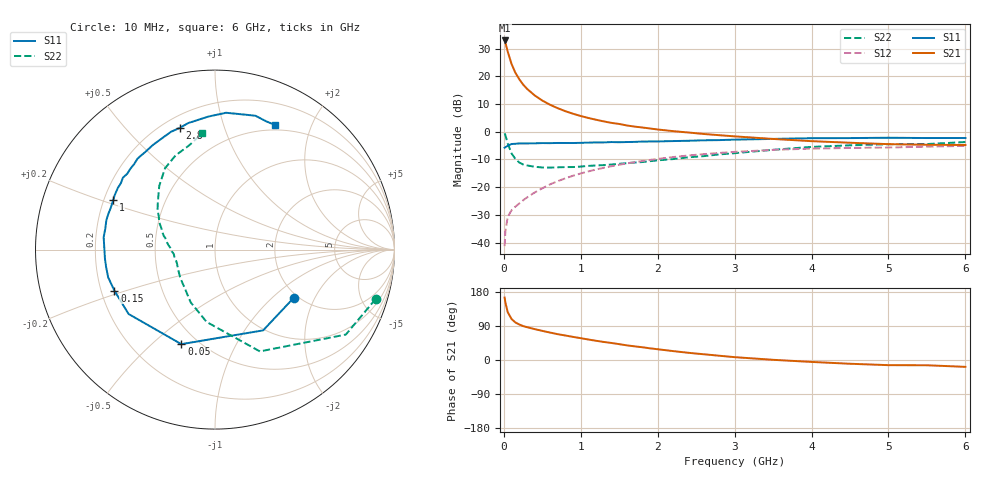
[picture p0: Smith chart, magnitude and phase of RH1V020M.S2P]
! SIEMENS Small Signal Semiconductors
! BFR106
! Si NPN RF Bipolar Junction Transistor in SOT23
! VCE = 1 V  IC = 20 mA
! Common Emitter S-Parameters:  August  1996
# GHz  S  MA  R  50
!  f  S11  S21  S12  S22
! GHz  MAG  ANG  MAG  ANG  MAG  ANG  MAG  ANG
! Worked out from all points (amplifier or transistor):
!   36 points, 10 MHz to 6 GHz, reference 50 ohm
!   highest |S21| = 33.0 dB at 10 MHz (marker M1)
!   |S21| within 3 dB of that: start of sweep to 40.81 MHz
!   unconditionally stable (mu >= 1): 332.5 MHz to 3.215 GHz; 4.097 GHz to end of sweep
!   at 250 MHz: K = 0.92, MSG = 20.9 dB, |S12| = -24.8 dB
!   at 1.4 GHz: K = 1.08, MAG = 6.0 dB, |S12| = -12.4 dB
!   at 6 GHz: K = 1.02, MAG = -0.8 dB, |S12| = -5.1 dB
!   S11 on the Smith chart (normalised r, x): 10 MHz: 1.89, -1.39; 50 MHz: 0.41, -0.62; 150 MHz: 0.25, -0.18; 1 GHz: 0.24, +0.22; 2.8 GHz: 0.27, +0.72; 6 GHz: 0.44, +1.50
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0.01  0.5142 -31.6  44.42 164.7  0.0086 79.8  0.9365 -17.1
0.02  0.5239 -59.2  40.78 152.0  0.0159 70.4  0.8692 -33.0
0.05  0.5592 -109.6  28.04 126.4  0.0291 51.9  0.6199 -66.2
0.1  0.6004 -143.3  16.75 108.1  0.0381 46.6  0.4059 -96.6
0.15  0.6053 -157.8  11.6 99.1  0.0445 49.0  0.3235 -114.8
0.2  0.6151 -165.5  8.879 93.8  0.0506 51.8  0.2787 -126.1
0.25  0.6143 -171.2  7.12 89.6  0.0578 54.4  0.2567 -136.0
0.3  0.6152 -175.3  5.975 86.7  0.0651 56.8  0.2469 -142.1
0.4  0.6177 178.2  4.535 81.5  0.0799 59.8  0.2331 -152.1
0.5  0.6242 173.6  3.652 76.9  0.0954 61.5  0.2263 -158.8
0.6  0.6223 169.2  3.071 72.4  0.1121 62.1  0.225 -163.0
0.7  0.6271 164.9  2.663 68.2  0.1281 62.0  0.228 -166.8
0.8  0.6267 161.6  2.347 64.6  0.1441 61.4  0.2301 -170.5
1  0.6305 154.2  1.922 57.6  0.1765 59.9  0.2349 -175.6
1.1  0.6362 151.2  1.77 54.0  0.1923 58.6  0.2418 -177.8
1.6  0.6519 136.3  1.297 38.6  0.2684 51.6  0.2708 171.3
2.2  0.6782 120.5  1.025 23.5  0.3491 41.9  0.3211 158.4
2.8  0.7061 106.1  0.866 11.3  0.4139 31.9  0.3896 145.2
3.5  0.742 92.9  0.741 0.5  0.4708 20.8  0.4722 131.1
4.5  0.7681 79.0  0.633 -9.9  0.5098 6.5  0.5689 112.7
5.5  0.7695 68.2  0.582 -13.9  0.5374 -2.2  0.5995 103.7
6  0.7707 64.2  0.576 -18.1  0.5552 -8.6  0.6516 96.2
